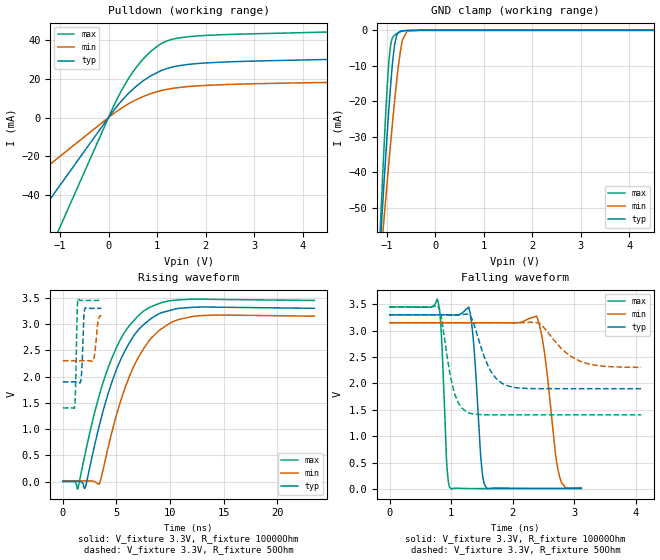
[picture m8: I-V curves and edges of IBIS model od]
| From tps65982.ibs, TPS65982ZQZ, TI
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|   od Model
[Model]   od
Model_type   Open_sink
Polarity   Non-Inverting
Vmeas = 1.65
Vref = 0
Cref = 2pF
Rref = 10000
|   typ   min   max
|   (nom PVT)   (fast PVT)   (slow PVT)
C_comp   2.678e-13   2.561e-13   2.882e-13
| Where nom  PVT is Nominal Process, 3.3V, 27C
|   Fast PVT is Strong Process,  3.45V, -40C
|   Slow PVT is Weak Process,   3.15V, 125C
[Voltage Range]   3.3   3.15   3.45
|Junction Temperature
[Temperature Range]   27   125   -40
[Pullup Reference]   3.3   3.15   3.45
[Pulldown Reference]   0   0   0
[Power Clamp Reference]   3.3   3.15   3.45
[GND Clamp Reference]   0   0   0
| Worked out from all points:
|   slope of the pulldown table from 0 to 0.495 V, typ, clamps not added: 34.3 ohm
|   GND clamp passes 1 mA (typ) near -0.78 V on its own axis
|   falling waveform, V_fixture 3.3V, R_fixture 10000Ohm: 20-80 % time 103ps typ, 175ps min, 71.3ps max; typ from 3.3 V to 0.009 V
|   rising waveform, V_fixture 3.3V, R_fixture 10000Ohm: 20-80 % time 3.27ns typ, 3.3ns min, 3.27ns max; typ from 0.009 V to 3.3 V
|   falling waveform, V_fixture 3.3V, R_fixture 50Ohm: 20-80 % time 274ps typ, 445ps min, 187ps max; typ from 3.3 V to 1.9 V
|   rising waveform, V_fixture 3.3V, R_fixture 50Ohm: 20-80 % time 157ps typ, 238ps min, 124ps max; typ from 1.9 V to 3.3 V
[Pulldown]
|   Voltage   I(typ)   I(min)   I(max)
-3.3V     -115.5mA   -66.05mA   -186.6mA
-150.2mV  -5.254mA   -3.005mA   -8.491mA
151.8mV   5.12mA     2.892mA    8.346mA
274.2mV   8.794mA    4.985mA    14.26mA
460.5mV   13.65mA    7.775mA    21.97mA
653.4mV   17.8mA     10.18mA    28.45mA
854.7mV   21.26mA    12.19mA    33.77mA
1.178V    25.09mA    14.42mA    39.29mA
1.422V    26.64mA    15.41mA    40.98mA
2.041V    28.23mA    16.63mA    42.43mA
5.432V    30.45mA    18.48mA    44.73mA
6.6V      31.82mA    19.33mA    46.75mA
[GND Clamp]
|   Voltage   I(typ)   I(min)   I(max)
-3.3V     -590.4mA   -444mA     -788.7mA
-1.199V   -74.63mA   -76.16mA   -75.51mA
-1.116V   -55.7mA    -62.46mA   -49.79mA
-1.076V   -46.71mA   -55.88mA   -37.81mA
-988.5mV  -28.1mA    -41.92mA   -14.79mA
-953.7mV  -21.22mA   -36.51mA   -8.034mA
-909.2mV  -13.21mA   -29.75mA   -3.193mA
-838.2mV  -3.917mA   -19.56mA   -1.317mA
-720.1mV  -245.2uA   -5.813mA   -406.6uA
-581.6mV  -16.32uA   -259.3uA   -33.6uA
-330mV    -28.52nA   -247.7nA   -18.68nA
6.6V      0A         0A         0A
[POWER Clamp]
|   Voltage   I(typ)   I(min)   I(max)
-3.3V     0A         0A         0A
0V        0A         0A         0A
6.6V      0A         0A         0A
[Ramp]
R_load = 10000
|   typ   min   max
dV/dt_r   1.97447/3.26362e-09   1.88062/3.29437e-09   2.06648/3.26666e-09
dV/dt_f   1.97447/1.03215e-10   1.88062/1.746e-10   2.06648/7.12696e-11
[Falling Waveform]
V_fixture = 3.3V
V_fixture_min = 3.15V
V_fixture_max = 3.45V
R_fixture = 10000Ohm
|   Time   V(typ)   V(min)   V(max)
0s        3.3V       3.15V      3.45V
778ps     3.3V       3.15V      3.586V
836ps     3.3V       3.15V      3.004V
922ps     3.3V       3.15V      579.2mV
974ps     3.298V     3.15V      32.6mV
1.308ns   3.328V     3.15V      6.451mV
1.536ns   96.46mV    3.15V      5.851mV
2.388ns   9.209mV    3.276V     5.867mV
2.762ns   9.201mV    226.3mV    5.867mV
3.114ns   9.21mV     24.24mV    5.866mV
[Rising Waveform]
V_fixture = 3.3V
V_fixture_min = 3.15V
V_fixture_max = 3.45V
R_fixture = 10000Ohm
|   Time   V(typ)   V(min)   V(max)
0s        9.212mV    15.64mV    5.866mV
1.088ns   9.21mV     15.64mV    3.455mV
1.388ns   9.243mV    15.64mV    -140.7mV
2.068ns   -123.2mV   15.63mV    521.4mV
3.392ns   1.062V     -43.35mV   1.642V
5.588ns   2.407V     1.661V     2.786V
7.538ns   2.991V     2.534V     3.25V
9.874ns   3.254V     3.003V     3.443V
12.06ns   3.318V     3.143V     3.477V
23.46ns   3.3V       3.151V     3.45V
[Falling Waveform]
V_fixture = 3.3V
V_fixture_min = 3.15V
V_fixture_max = 3.45V
R_fixture = 50Ohm
|   Time   V(typ)   V(min)   V(max)
0s        3.3V       3.15V      3.45V
780ps     3.3V       3.15V      3.471V
838ps     3.3V       3.15V      3.264V
1.034ns   3.299V     3.15V      1.895V
1.252ns   3.315V     3.15V      1.46V
1.63ns    2.259V     3.15V      1.405V
1.926ns   1.95V      3.15V      1.405V
2.41ns    1.901V     3.149V     1.405V
3.182ns   1.9V       2.386V     1.405V
4.088ns   1.9V       2.304V     1.405V
[Rising Waveform]
V_fixture = 3.3V
V_fixture_min = 3.15V
V_fixture_max = 3.45V
R_fixture = 50Ohm
|   Time   V(typ)   V(min)   V(max)
0s        1.9V       2.304V     1.405V
1.09ns    1.9V       2.304V     1.426V
1.172ns   1.9V       2.304V     1.701V
1.322ns   1.901V     2.304V     3.12V
1.408ns   1.9V       2.304V     3.471V
1.722ns   2.001V     2.304V     3.45V
2.02ns    3.266V     2.304V     3.45V
2.888ns   3.3V       2.341V     3.45V
3.274ns   3.3V       3.041V     3.45V
3.598ns   3.3V       3.15V      3.45V
